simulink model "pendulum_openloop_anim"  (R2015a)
settings: Solver=ode45  StartTime=0.0  StopTime=100  RelTol=1e-3
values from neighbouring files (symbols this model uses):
  g = 9.81    [pendulum_sys_init.m]
  kc = 2    [pendulum_sys_init.m]
  ke = 2    [pendulum_sys_init.m]
  l = 1    [pendulum_sys_init.m]
  M = 10    [pendulum_sys_init.m]
  m = 2    [pendulum_sys_init.m]
  ra = 10    [pendulum_sys_init.m]
  rr = .1    (= 0.1)    [pendulum_sys_init.m]
undefined symbols (not defined in the file or in its folder): pendolo_sys_diff
libraries: simulink x1, vrlib x1

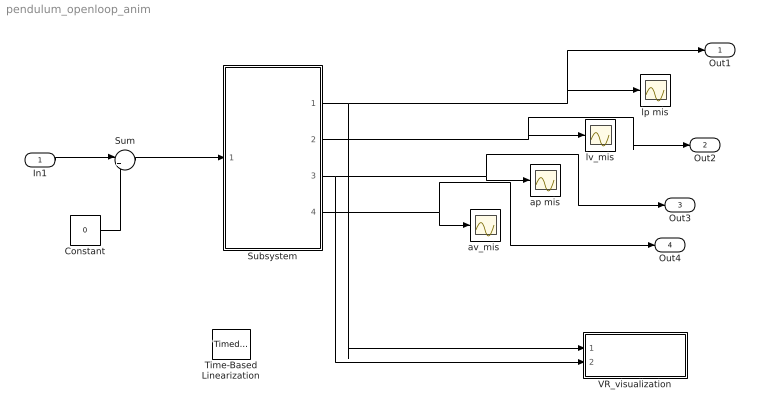
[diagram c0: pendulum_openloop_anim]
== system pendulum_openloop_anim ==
  In1 : Inport
  Constant : Constant  Value=0
  Subsystem : Subsystem
  Sum : Sum  Inputs=|++
  Time-Based Linearization : simulink/Model-Wide Utilities/Timed-Based Linearization  LinearizationTime=1  SampleTime=0
  VR_visualization : Subsystem
  ap mis : Scope
  "av_mis " : Scope
  lp mis : Scope
  lv_mis : Scope
  Out1 : Outport
  Out2 : Outport  Port=2
  Out3 : Outport  Port=3
  Out4 : Outport  Port=4
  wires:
  Subsystem/3(ap) -> VR_visualization/2(ap), Out3/1, ap mis/1
  Subsystem/1(lp) -> VR_visualization/1(lp), Out1/1, lp mis/1
  Subsystem/2(lv) -> Out2/1, lv_mis/1
  Subsystem/4(av) -> Out4/1, "av_mis "/1
  In1/1 -> Sum/1
  Constant/1 -> Sum/2
  Sum/1 -> Subsystem/1(voltage)

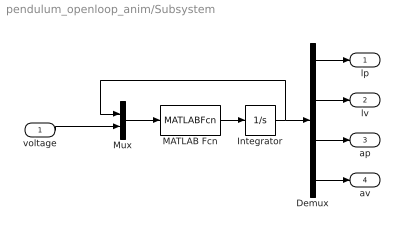
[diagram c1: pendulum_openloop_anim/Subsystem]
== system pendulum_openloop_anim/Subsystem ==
  voltage : Inport
  Demux : Demux
  Integrator : Integrator  InitialCondition=[0 0.0 0 0]
  MATLAB Fcn : MATLABFcn  MATLABFcn=pendolo_sys_diff(u,M,m,l,ra,rr,ke,kc,g)
  Mux : Mux  Inputs=2
  lp : Outport
  lv : Outport  Port=2
  ap : Outport  Port=3
  av : Outport  Port=4
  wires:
  MATLAB Fcn/1 -> Integrator/1
  Integrator/1 -> Demux/1, Mux/1
  Demux/4 -> av/1
  Demux/3 -> ap/1
  Demux/2 -> lv/1
  Demux/1 -> lp/1
  Mux/1 -> MATLAB Fcn/1
  voltage/1 -> Mux/2

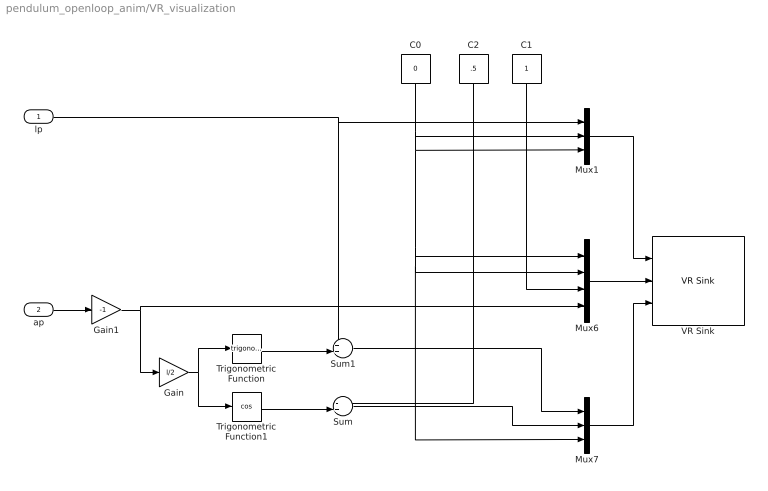
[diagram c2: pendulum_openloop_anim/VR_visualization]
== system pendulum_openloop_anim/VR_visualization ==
  lp : Inport
  ap : Inport  Port=2
  C0 : Constant  Value=0
  C1 : Constant
  C2 : Constant  Value=.5
  Gain : Gain  Gain=l/2
  Gain1 : Gain  Gain=-1
  Mux1 : Mux  Inputs=3
  Mux6 : Mux
  Mux7 : Mux  Inputs=3
  Sum : Sum  Inputs=-+|
  Sum1 : Sum  Inputs=++|
  Trigonometric Function : Trigonometry
  Trigonometric Function1 : Trigonometry  Operator=cos
  VR Sink : vrlib/VR Sink  InstantiateOnLoad=on  SampleTime=0.02  ViewEnable=on  RemoteChange=off  RemoteView=off  FieldsWritten=carrello.translation.3.1.double#asta.rotation.4.1.double#asta.translation.3.1.double  WorldFileName=vrml1.wrl  AutoView=on  VideoDimensions=[]  AllowVariableSize=off
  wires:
  Mux1/1 -> VR Sink/1
  Mux6/1 -> VR Sink/2
  Mux7/1 -> VR Sink/3
  lp/1 -> Mux1/1, Sum1/1
  C0/1 -> Mux1/2, Mux1/3, Mux6/1, Mux6/2, Mux7/3
  ap/1 -> Gain1/1
  C1/1 -> Mux6/3
  Trigonometric Function/1 -> Sum1/2
  Trigonometric Function1/1 -> Sum/2
  Sum1/1 -> Mux7/1
  Sum/1 -> Mux7/2
  C2/1 -> Sum/1
  Gain/1 -> Trigonometric Function/1, Trigonometric Function1/1
  Gain1/1 -> Mux6/4, Gain/1
